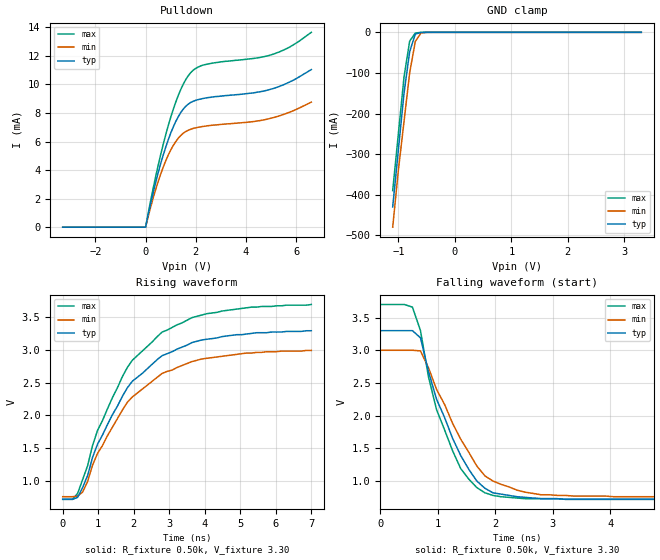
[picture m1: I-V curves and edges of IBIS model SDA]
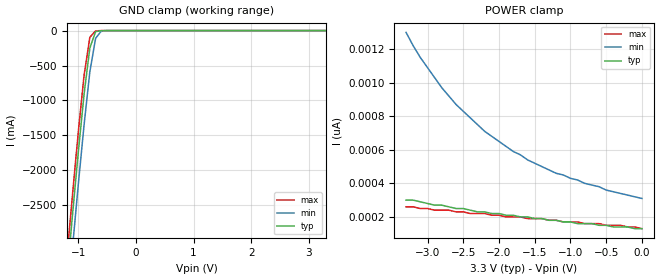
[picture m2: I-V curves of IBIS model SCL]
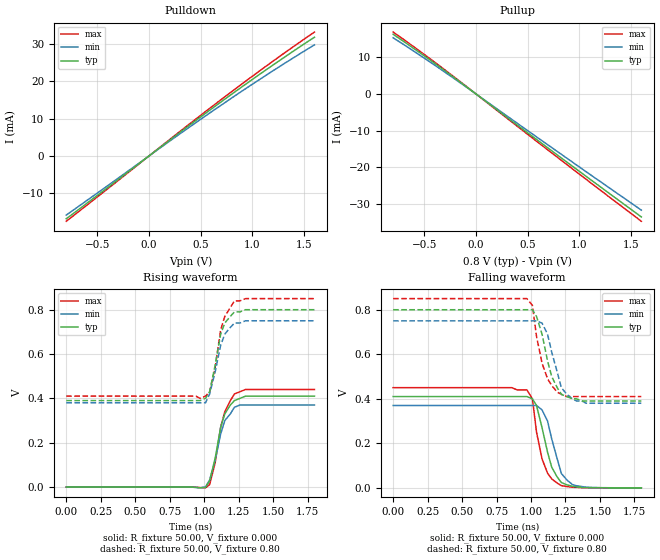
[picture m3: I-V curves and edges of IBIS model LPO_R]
| Integrated Devices Technolgy, Inc
[Ibis Ver]   3.2
[File Name]   9lrs3187.ibs
[File Rev]   1.4
|06/18/2009 Rev 1.0 created by wm
|08/26/2009 Rev 1.1 Rref resistor values edited on output drivers.
|11/10/2009 Rev 1.2 Corrected LPO_R model
|05/05/2010 Rev 1.3 Added rev B component.  Changed to model selector for SE.
|09/25/2013 1.4 Corrected SCL model
[Date]   09/26/2013
[Source]   Integrated Devices Technolgy, Inc.
[Notes]   Rev 0.0 created by wm
[Disclaimer] Integrated Device Technology, Inc. ("IDT") hereby grants the
   user of this IBIS model a non-exclusive, nontransferable
   license to use this IBIS model under the following terms. The
   user is granted this license only to use the IBIS model and is
   not granted rights to sell, copy (except as needed to run the
   IBIS model), rent, lease or sub-license the IBIS model in
   whole or in part, or in modified form to anyone. The User may
   modify the IBIS model to suit its specific applications, but
   rights to derivative works and such modifications shall belong
   to IDT. This IBIS model is provided on an AS IS" basis and IDT
   makes absolutely no warranty with respect to the information
   contained herein. IDT DISCLAIMS AND CUSTOMER WAIVES ALL
   WARRANTIES, EXPRESS AND IMPLIED, INCLUDING WARRANTIES OF
   MERCHANTABILITY AND FITNESS FOR A PARTICULAR PURPOSE. THE
   ENTIRE RISK AS TO QUALITY AND PERFORMANCE IS WITH THE USER
   ACCORDINGLY, IN NO EVENT SHALL IDT BE LIABLE FOR ANY DIRECT OR
   INDIRECT DAMAGES, WHETHER IN CONTRACT OR TORT, INCLUDING ANY
   LOST PROFITS OR OTHER INCIDENTAL, CONSEQUENTIAL, EXEMPLARY, OR
   PUNITIVE DAMAGES ARISING OUT OF THE USE OR APPLICATION OF THE
   IBIS model. Further, IDT reserves the right to make changes
   without notice to any product herein to improve reliability,
   function, or design. IDT does not convey any license under
   patent rights or any other intellectual property rights,
   including those of third parties. IDT is not obligated to
   provide maintenance or support for the licensed IBIS model.
[Copyright]   Copyright 2006, Integrated Devices Technolgy, Inc. all rights
   reserved
|   COMPONENT: ICS9LRS3187A
[Component]   IDT9LRS3187A
[Manufacturer]   Integrated Device Technology, Inc.
[Package]
| variable   typ   min   max
R_pkg   81.1m   62.2m   100.0m
L_pkg   6.7nH   4.9nH   8.5nH
C_pkg   0.53pF   0.21pF   0.85pF
[Pin]  signal_name   model_name   R_pin   L_pin   C_pin
1   VDD96   POWER
2   GND96   GND
3   DOTT96   LPO_R
4   DOTC96   LPO_R
5   VDD27M   POWER
6   27MHz_NonSS   SE_2X_SR
7   27MHz_SS   SE_2X_SR
8   GND27M   GND
9   GNDSATA   GND
10   SATAT   LPO_R
11   SATAC   LPO_R
12   GNDSRC   GND
13   SRCT1   LPO_R
14   SRCC1   LPO_R
15   VDDSRC_IO   POWER
16   CPU_STOP#   IN
17   VDDSRC   POWER
18   VDDCPU_IO   POWER
19   CPUC1   LPO_R
20   CPUT1   LPO_R
21   GNDCPU   GND
22   CPUC0   LPO_R
23   CPUT0   LPO_R
24   VDDCPU   POWER
25   CK_PWRGD/PD#   IN
26   GNDREF   GND
27   X2   XTL_OUT
28   X1   XT1
29   VDDREF   POWER
30   FSLC/REF0   SE_2X_SR_LVIN_IO
31   SDATA   SDA
32   SCLK   SCL
[Diff Pin]   inv_pin   vdiff   tdelay_typ   tdelay_min   tdelay_max
3   4   NA   NA
10   11   NA   NA
13   14   NA   NA
20   19   NA   NA
23   22   NA   NA
[Model Selector] SE_2X_SR
SE_2X_SR_115   Slew = 1V/ns
SE_2X_SR_192   Slew = 2V/ns.
[Model Selector] SE_2X_SR_LVIN_IO
SE_2X_SR_115_LVIN_IO   Slew = 1V/ns
SE_2X_SR_192_LVIN_IO   Slew = 2V/ns.
|   COMPONENT: ICS9LRS3187B
[Component]   IDT9LRS3187B
[Manufacturer]   Integrated Device Technology, Inc.
[Package]
| variable   typ   min   max
R_pkg   81.1m   62.2m   100.0m
L_pkg   6.7nH   4.9nH   8.5nH
C_pkg   0.53pF   0.21pF   0.85pF
[Pin]  signal_name   model_name   R_pin   L_pin   C_pin
1   VDD96   POWER
2   GND96   GND
3   DOTT96   LPO_R
4   DOTC96   LPO_R
5   VDD27M   POWER
6   27MHz_NonSS   SE_2X_SR
7   27MHz_SS   SE_2X_SR
8   GND27M   GND
9   GNDSATA   GND
10   SATAT   LPO_R
11   SATAC   LPO_R
12   GNDSRC   GND
13   SRCT1   LPO_R
14   SRCC1   LPO_R
15   VDDSRC_IO   POWER
16   CPU_STOP#   IN
17   VDDSRC   POWER
18   VDDCPU_IO   POWER
19   CPUC1   LPO_R
20   CPUT1   LPO_R
21   GNDCPU   GND
22   CPUC0   LPO_R
23   CPUT0   LPO_R
24   VDDCPU   POWER
25   CK_PWRGD/PD#   IN
26   GNDREF   GND
27   X2   XTL_OUT
28   X1   XT1
29   VDDREF   POWER
30   FSLC/REF0   SE_2X_SR_LVIN_IO
31   SDATA   SDA
32   SCLK   SCL
[Diff Pin]   inv_pin   vdiff   tdelay_typ   tdelay_min   tdelay_max
3   4   NA   NA
10   11   NA   NA
13   14   NA   NA
20   19   NA   NA
23   22   NA   NA
| Models and submodels in the file (10): SDA (I/O_open_drain), SCL (Input), LPO_R (Output), XT1 (Input), IN (Input), XTL_OUT (Output), SE_2X_SR_115 (Output), SE_2X_SR_192 (Output), SE_2X_SR_115_LVIN_IO (I/O), SE_2X_SR_192_LVIN_IO (I/O)
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|   Model SDA
[Model]   SDA
Model_type   I/O_open_drain
Polarity   Inverting
Enable   Active-High
Vinl =   0.80V
Vinh =   2.00V
Vmeas =   1.50V
Cref =   5.00pF
Vref =   1.50V
Rref =   500
C_comp   3.40pF   2.85pF   3.95pF
[Temperature Range]   27.00   70.00   0.000
[Voltage Range]   3.30V   3.00V   3.70V
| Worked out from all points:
|   slope of the pulldown table from 0 to 0.495 V, typ, clamps not added: 131 ohm
|   GND clamp passes 1 mA (typ) near -0.62 V on its own axis
|   rising waveform, R_fixture 0.50k, V_fixture 3.30: 20-80 % time 1.74ns typ, 1.76ns min, 1.73ns max; typ from 0.72 V to 3.29 V
|   falling waveform, R_fixture 0.50k, V_fixture 3.30: 20-80 % time 693ps typ, 785ps min, 596ps max; typ from 3.3 V to 0.72 V
[Pulldown]
| voltage   I(typ)   I(min)   I(max)
-3.3V     0A         0A         0A
0V        0A         0A         0A
500mV     3.8mA      3.19mA     4.32mA
900mV     6.11mA     5.04mA     7.1mA
1.2V      7.4mA      5.99mA     8.75mA
1.4V      8.03mA     6.42mA     9.64mA
1.8V      8.74mA     6.86mA     10.83mA
2.1V      8.94mA     7mA        11.22mA
2.5V      9.08mA     7.11mA     11.44mA
5.1V      9.72mA     7.68mA     12.13mA
5.7V      10.14mA    8.03mA     12.58mA
6.6V      11.04mA    8.76mA     13.65mA
[GND_clamp]
| voltage   I(typ)   I(min)   I(max)
  |-3.30   -3.78A   -3.64A   -3.87A
  |-3.20   -3.62A   -3.50A   -3.71A
  |-3.10   -3.47A   -3.35A   -3.55A
  |-3.00   -3.31A   -3.21A   -3.39A
  |-2.90   -3.16A   -3.06A   -3.23A
  |-2.80   -3.01A   -2.91A   -3.07A
  |-2.70   -2.85A   -2.77A   -2.91A
  |-2.60   -2.70A   -2.62A   -2.75A
  |-2.50   -2.54A   -2.48A   -2.59A
  |-2.40   -2.39A   -2.33A   -2.43A
  |-2.30   -2.24A   -2.19A   -2.27A
  |-2.20   -2.08A   -2.04A   -2.11A
  |-2.10   -1.93A   -1.90A   -1.95A
  |-2.00   -1.78A   -1.75A   -1.79A
  |-1.90   -1.62A   -1.61A   -1.63A
  |-1.80   -1.47A   -1.46A   -1.47A
  |-1.70   -1.32A   -1.32A   -1.32A
  |-1.60   -1.17A   -1.18A   -1.16A
  |-1.50   -1.02A   -1.03A   -1.00A
  |-1.40   -0.87A   -0.89A   -0.85A
  |-1.30   -0.72A   -0.75A   -0.69A
  |-1.20   -0.57A   -0.61A   -0.54A
-1.1V     -430mA     -480mA     -390mA
-1V       -290mA     -340mA     -250mA
-900mV    -150mA     -220mA     -110mA
-800mV    -47.73mA   -100mA     -21.74mA
-700mV    -4.4mA     -22.46mA   -1.7mA
-600mV    -390uA     -1.82mA    -190uA
-400mV    -1.59uA    -9.25uA    -420nA
3.3V      150pA      220pA      150pA
[Ramp]
| variable   typ   min   max
dV/dt_r   0.27/0.19n   0.21/0.19n   0.35/0.18n
dV/dt_f   0.27/0.21n   0.21/0.22n   0.35/0.20n
[Rising Waveform]
R_fixture = 0.50k
V_fixture = 3.30
V_fixture_min = 3.00
V_fixture_max = 3.70
| time   V(typ)   V(min)   V(max)
0s        720mV      760mV      720mV
280ps     720mV      760mV      720mV
420ps     750mV      770mV      810mV
560ps     900mV      830mV      1.02V
700ps     1.08V      990mV      1.23V
980ps     1.56V      1.42V      1.77V
1.82ns    2.42V      2.2V       2.73V
2.8ns     2.91V      2.64V      3.27V
4.06ns    3.16V      2.87V      3.55V
7ns       3.29V      2.99V      3.69V
[Falling Waveform]
R_fixture = 0.50k
V_fixture = 3.30
V_fixture_min = 3.00
V_fixture_max = 3.70
| time   V(typ)   V(min)   V(max)
0s        3.3V       3V         3.7V
560ps     3.3V       3V         3.66V
700ps     3.19V      2.99V      3.3V
840ps     2.67V      2.73V      2.59V
980ps     2.25V      2.4V       2.09V
1.4ns     1.39V      1.64V      1.19V
1.68ns    1V         1.23V      900mV
1.82ns    890mV      1.08V      820mV
2.8ns     730mV      790mV      730mV
7ns       720mV      760mV      720mV
|   Model SCL
[Model]   SCL
Model_type   Input
Polarity   Inverting
Vinl =   0.80V
Vinh =   2.00V
C_comp   3.40pF   2.85pF   3.95pF
[Temperature Range]   27.00   70.00   0.000
[Voltage Range]   3.30V   3.00V   3.70V
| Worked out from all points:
|   GND clamp passes 1 mA (typ) near -0.60 V on its own axis
[GND_clamp]
| voltage   I(typ)   I(min)   I(max)
-3.3V     -24.05A    -24.49A    -23.79A
-1.2V     -3.55A     -4.02A     -3.26A
-1.1V     -2.63A     -3.1A      -2.34A
-1V       -1.74A     -2.2A      -1.45A
-900mV    -910mA     -1.35A     -640mA
-800mV    -250mA     -590mA     -96.82mA
-700mV    -14.58mA   -110mA     -3.87mA
-600mV    -880uA     -5.84mA    -450uA
-500mV    -88.5uA    -350uA     -45.09uA
3.3V      130pA      340pA      120pA
[POWER_clamp]
| voltage   I(typ)   I(min)   I(max)
-3.3V     300pA      1.3nA      260pA
-3.1V     290pA      1.15nA     250pA
-2.9V     270pA      1.03nA     240pA
-2.8V     270pA      970pA      240pA
-2.6V     250pA      870pA      230pA
-2.2V     230pA      710pA      220pA
-1.8V     210pA      590pA      200pA
-1.2V     180pA      460pA      180pA
-900mV    160pA      420pA      170pA
-500mV    150pA      360pA      150pA
-300mV    140pA      340pA      150pA
0V        130pA      310pA      130pA
|   Model LPO_R   V2
[Model]   LPO_R
Model_type   Output
Polarity   Inverting
Vmeas  =  0.4V
C_comp   3.40pF   2.85pF   3.95pF
[Temperature Range]   27.00   70.00   0.000
[Voltage Range]   0.80V   0.75V   0.85V
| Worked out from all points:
|   slope of the pulldown table from 0 to 0.12 V, typ, clamps not added: 47.2 ohm
|   slope of the pullup table from 0 to 0.12 V, typ, clamps not added: 47 ohm
|   rising waveform, R_fixture 50.00, V_fixture 0.000: 20-80 % time 87.8ps typ, 89ps min, 88.5ps max; typ from 0 V to 0.41 V
|   rising waveform, R_fixture 50.00, V_fixture 0.80: 20-80 % time 82.8ps typ, 88ps min, 81.3ps max; typ from 0.39 V to 0.8 V
|   falling waveform, R_fixture 50.00, V_fixture 0.000: 20-80 % time 103ps typ, 94.1ps min, 86.9ps max; typ from 0.41 V to 0 V
|   falling waveform, R_fixture 50.00, V_fixture 0.80: 20-80 % time 106ps typ, 93ps min, 93ps max; typ from 0.8 V to 0.39 V
[Pulldown]
| voltage   I(typ)   I(min)   I(max)
-800mV    -16.76mA   -15.78mA   -17.43mA
600mV     12.47mA    11.71mA    12.99mA
1.1V      22.38mA    20.97mA    23.32mA
1.6V      31.7mA     29.66mA    33.08mA
[Pullup]
| voltage   I(typ)   I(min)   I(max)
-800mV    16.2mA     15.25mA    16.8mA
-300mV    6.28mA     5.91mA     6.52mA
700mV     -14.78mA   -13.94mA   -15.33mA
1.6V      -33.46mA   -31.61mA   -34.64mA
[Ramp]
| variable   typ   min   max
dV/dt_r   0.25/88.04p   0.22/90.43p   0.27/84.29p
dV/dt_f   0.25/89.71p   0.22/94.68p   0.27/86.85p
R_load = 50.00
[Rising Waveform]
R_fixture = 50.00
V_fixture = 0.000
V_fixture_min = 0.000
V_fixture_max = 0.000
| time   V(typ)   V(min)   V(max)
0s        0V         0V         0V
1.01ns    -1.57mV    620uV      -3.6mV
1.04ns    28.04mV    32.36mV    11.03mV
1.08ns    130mV      120mV      110mV
1.12ns    270mV      240mV      270mV
1.15ns    330mV      300mV      340mV
1.19ns    370mV      330mV      390mV
1.22ns    390mV      360mV      420mV
1.3ns     410mV      370mV      440mV
1.8ns     410mV      370mV      440mV
[Rising Waveform]
R_fixture = 50.00
V_fixture = 0.80
V_fixture_min = 0.75
V_fixture_max = 0.85
| time   V(typ)   V(min)   V(max)
0s        390mV      380mV      410mV
940ps     390mV      380mV      410mV
970ps     390mV      380mV      400mV
1.01ns    400mV      380mV      410mV
1.04ns    430mV      420mV      430mV
1.08ns    550mV      520mV      540mV
1.12ns    690mV      640mV      710mV
1.15ns    740mV      690mV      770mV
1.22ns    790mV      740mV      840mV
1.8ns     800mV      750mV      850mV
[Falling Waveform]
R_fixture = 50.00
V_fixture = 0.000
V_fixture_min = 0.000
V_fixture_max = 0.000
| time   V(typ)   V(min)   V(max)
0s        410mV      370mV      450mV
970ps     410mV      370mV      440mV
1.01ns    400mV      370mV      400mV
1.04ns    370mV      370mV      250mV
1.08ns    270mV      350mV      130mV
1.12ns    160mV      300mV      65.86mV
1.15ns    92.88mV    220mV      40.16mV
1.22ns    23.85mV    64.57mV    9.99mV
1.3ns     7.09mV     14.76mV    2.7mV
1.8ns     72.44uV    110uV      52.48uV
[Falling Waveform]
R_fixture = 50.00
V_fixture = 0.80
V_fixture_min = 0.75
V_fixture_max = 0.85
| time   V(typ)   V(min)   V(max)
0s        800mV      750mV      850mV
970ps     800mV      750mV      850mV
1.01ns    800mV      750mV      820mV
1.04ns    770mV      750mV      680mV
1.08ns    690mV      740mV      560mV
1.15ns    500mV      610mV      460mV
1.19ns    450mV      520mV      430mV
1.22ns    420mV      450mV      420mV
1.33ns    400mV      390mV      410mV
1.8ns     390mV      380mV      410mV
